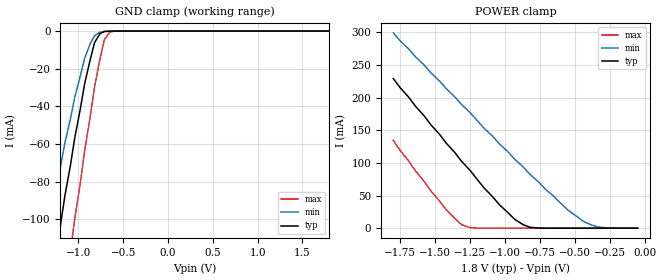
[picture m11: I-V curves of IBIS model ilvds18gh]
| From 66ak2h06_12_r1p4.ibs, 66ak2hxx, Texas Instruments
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|   Model Cell ilvds18gh
|   Model Cell ilvds18gh
|ilvds18gh.ibs   [11Jan12 revision 1.0]
[Model]   ilvds18gh
Model_type   Input
Polarity   Non-Inverting
Vinl =  1.15
Vinh =  1.25
C_comp   0.824869p   0.789813p   0.848489p
[Model Spec]
Vinl   1.15   1.15   1.15
Vinh   1.25   1.25   1.25
[Temperature Range]   25   125   -40
[Voltage Range]   1.8   1.62   1.98
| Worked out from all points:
|   GND clamp passes 1 mA (typ) near -0.74 V on its own axis
|   POWER clamp passes 1 mA (typ) near -0.81 V on its own axis
[GND_clamp]
|   voltage   I(typ)   I(min)   I(max)
-1.8V     -284.5mA   -222mA     -365.6mA
-1.36V    -151.8mA   -111.8mA   -212.1mA
-1.31V    -135.5mA   -98.36mA   -193.1mA
-1.2V     -103.3mA   -72.11mA   -155.3mA
-1.09V    -71.8mA    -46.98mA   -117.9mA
-1.04V    -56.54mA   -35.13mA   -99.51mA
-930mV    -27.93mA   -14.42mA   -63.46mA
-820mV    -6.162mA   -2.468mA   -29.72mA
-760mV    -1.428mA   -681.2uA   -15.1mA
-710mV    -221.1uA   -161.8uA   -4.512mA
-600mV    -3.7uA     -7.577uA   -45.99uA
1.8V      756.9pA    232.1nA    158.3pA
[POWER_clamp]
|   voltage   I(typ)   I(min)   I(max)
-1.8V     229.3mA    299.2mA    134.7mA
-1.53V    158.2mA    237.9mA    56.74mA
-1.42V    130mA      213.5mA    27.87mA
-1.31V    102.2mA    189.2mA    5.191mA
-1.25V    88.46mA    177.1mA    777.8uA
-1.04V    35.83mA    129.1mA    98.12nA
-870mV    5.306mA    93.75mA    34.49nA
-760mV    196.5uA    70.75mA    19.16nA
-550mV    58.7nA     27.8mA     4.967nA
-440mV    5.283nA    10.54mA    2.323nA
-330mV    2.472nA    1.6mA      1.055nA
-50mV     847.2pA    1.03uA     200.1pA
